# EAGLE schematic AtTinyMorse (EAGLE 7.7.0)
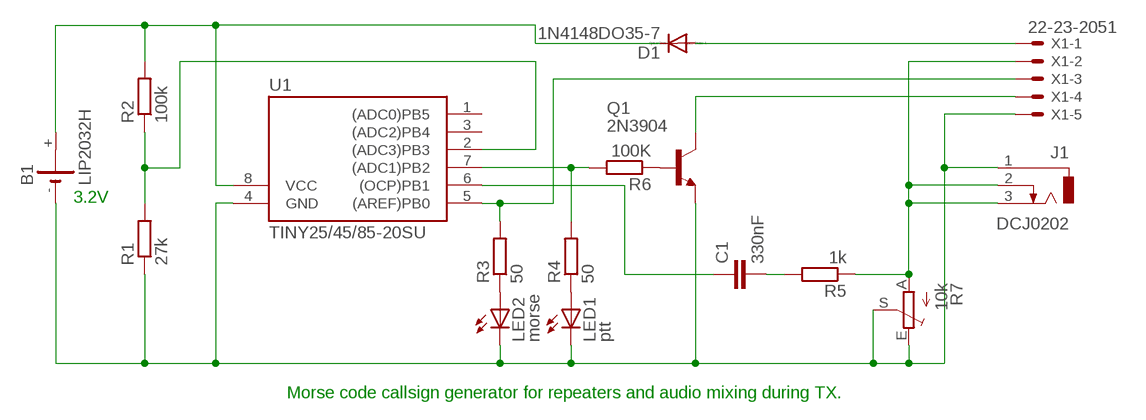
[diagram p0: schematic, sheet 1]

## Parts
B1  LIP2032H  CR2032H  [CR2032H]
C1  330nF  C5/2.5  [C5B2.5]
D1  1N4148DO35-7  [DO35-7]
J1  DCJ0202  [DCJ0202]
LED1  ptt  LED3MM  [LED3MM]
LED2  morse  LED3MM  [LED3MM]
Q1  2N3904  [TO92]
R1  27k  R-EU_0204/7  [0204/7]
R2  100k  R-EU_0204/7  [0204/7]
R3  50  R-EU_0204/7  [0204/7]
R4  50  R-EU_0204/7  [0204/7]
R5  1k  R-EU_0204/7  [0204/7]
R6  100K  R-EU_0204/7  [0204/7]
R7  10k  TRIM_EU-LI10  [LI10]
U1  TINY25/45/85-20SU  [SOIC8]
X1  22-23-2051  [22-23-2051]

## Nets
N$1: LED2.A R3.1
N$2: LED1.A R4.1
N$3: B1.- J1.1 LED1.K(C) LED2.K(C) Q1.3(E) R1.1 R7.E R7.S U1.4(GND) X1.5
N$4: Q1.1(C) X1.4
N$5: B1.+ D1.C R2.2 U1.8(VCC)
N$6: R1.2 R2.1 U1.2((ADC3)PB3)
N$7: C1.1 U1.6((OCP)PB1)
N$8: R3.2 U1.5((AREF)PB0) X1.3
N$9: C1.2 R5.2
N$10: J1.2 J1.3 R5.1 R7.A X1.2
N$11: R4.2 R6.2 U1.7((ADC1)PB2)
N$12: Q1.2(B) R6.1
N$13: D1.A X1.1
Unconnected: B1.+@1(+) U1.1((ADC0)PB5) U1.3((ADC2)PB4)

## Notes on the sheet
- 3.2V
- Morse code callsign generator for repeaters and audio mixing during TX.

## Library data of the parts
B1 = battery:CR2032H: LI BATTERY Varta
C1 = capacitor-wima:C: CAPACITOR
D1 = diode:1N4148: DIODE
J1 = con-jack:DCJ0202: DC POWER JACK Source: DCJ0202.pdf; OC_FARNELL: unknown; OC_NEWARK: unknown
LED1 LED2 = led:LED: LED
Q1 = transistor-npn:2N3904: NPN Transistor
R1-R6 = resistor:R-EU_: RESISTOR, European symbol
R7 = pot:TRIM_EU-: POTENTIOMETER
U1 = avr-7:TINY25/45/85
X1 = con-molex:22-23-2051: .100" (2.54mm) Center Header - 5 Pin; MF: MOLEX; MPN: 22-23-2051; OC_FARNELL: 1462952; OC_NEWARK: 38C9178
